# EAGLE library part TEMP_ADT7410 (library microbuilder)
ADT7410 - 13-bit 0.5°C I2C Temperature Sensor Operating Voltage: 2.7-5.5V Temperature Range: -55°C-150°C Accuracy: 0.5°C from -40°C-105°C Shutdown Current: 2uA (3.3V) Typical Operating Current (1 Sample/s): 46uA (3.3V) Digikey: ADT7410TRZ-ND
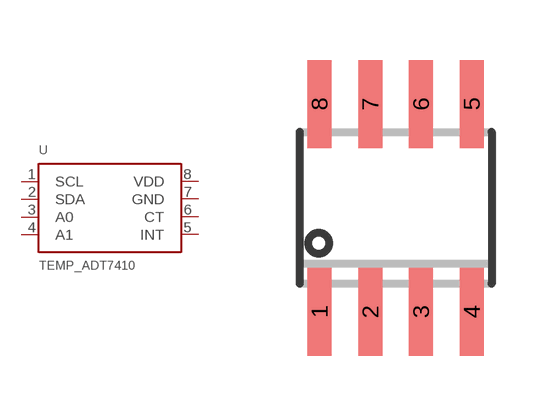
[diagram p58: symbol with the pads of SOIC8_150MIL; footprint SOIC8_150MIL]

Designator prefix U

## TEMP_ADT7410  [SOIC8_150MIL]
1  SCL
2  SDA
3  A0
4  A1
5  INT
6  CT
7  GND  pwr
8  VDD  pwr

## Footprint SOIC8_150MIL (pad centres in mm)
Small Outline IC - 150mil Wide
smd 0.6 x 2.2: 1 -1.905,-2.6; 2 -0.635,-2.6; 3 0.635,-2.6; 4 1.905,-2.6; 5 1.905,2.6; 6 0.635,2.6; 7 -0.635,2.6; 8 -1.905,2.6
